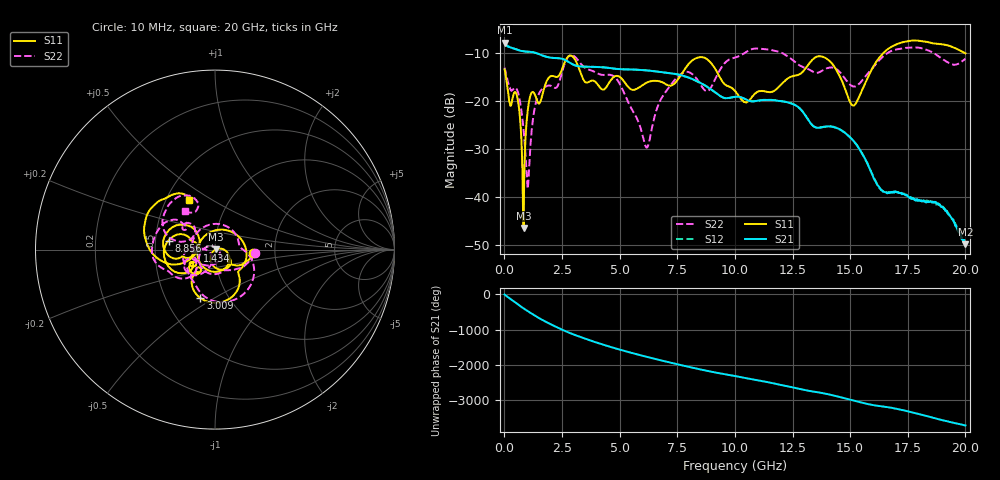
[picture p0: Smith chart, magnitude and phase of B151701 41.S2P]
!  2-Port S-parameters saved by WinCal
! VAR MeasName=S-Parameters (CALIBRATED_DATA) read from VNA (N5244A)
! VAR MeasDate=2015-12-24 19:14:13
! VAR NAME=B151701 41
! VAR FILENAME=B151701 41.S2P
! VAR DATE=2015-12-24 19:14:13
! VAR PHYS_PORTS=1,3
# Hz S DB R 50
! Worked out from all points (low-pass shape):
!   801 points, 10 MHz to 20 GHz, reference 50 ohm
!   highest |S21| = -7.85 dB at 10 MHz (marker M1); lowest = -49.8 dB at 20 GHz (marker M2)
!   |S21| within 3 dB of the highest: start of sweep to 1.852 GHz
!   lowest |S11| = -46.4 dB at 834.6 MHz (marker M3), VSWR 1.01, Z = 50.5 + j0.0707 ohm
!   |S11| at or under -10 dB: start of sweep to 16.45 GHz; 19.97049 GHz to end of sweep
!   |S22| runs from -38.2 to -8.9 dB; largest |S21 - S12| = 0.0028
!   S11 on the Smith chart (normalised r, x): 10 MHz: 1.54, -0.06; 1.434 GHz: 0.82, -0.01; 3.009 GHz: 0.74, -0.43; 8.856 GHz: 0.59, +0.06; 20 GHz: 0.65, +0.40
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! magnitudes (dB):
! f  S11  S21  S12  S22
! 10 MHz  -13.4  -7.8  -7.8  -13.1
! 234.9 MHz  -20.4  -8.8  -8.8  -17.2
! 559.7 MHz  -19.2  -9.4  -9.3  -17.8
! 834.6 MHz  -46.4  -9.7  -9.7  -26.1
! 1.034 GHz  -21.1  -9.8  -9.7  -37.2
! 1.434 GHz  -20.1  -10.1  -10.1  -19.2
! 3.009 GHz  -11.0  -12.5  -12.5  -10.6
! 3.358 GHz  -14.8  -12.8  -12.8  -12.5
! 4.283 GHz  -17.6  -13.0  -13.0  -14.6
! 4.883 GHz  -14.8  -13.3  -13.3  -15.5
! 6.157 GHz  -16.2  -13.6  -13.6  -29.7
! 6.682 GHz  -15.9  -13.9  -13.9  -20.7
! 7.806 GHz  -13.5  -14.8  -14.8  -14.0
! 8.856 GHz  -11.6  -17.2  -17.2  -17.8
! 10.01 GHz  -17.9  -19.1  -19.1  -11.0
! 11.65 GHz  -18.0  -19.8  -19.8  -9.5
! 13.35 GHz  -11.5  -25.0  -25.0  -13.8
! 14.15 GHz  -11.9  -25.3  -25.2  -13.0
! 15.15 GHz  -21.0  -28.4  -28.4  -17.0
! 16.68 GHz  -9.1  -39.0  -38.9  -9.9
! 18.95 GHz  -8.2  -42.0  -41.7  -11.1
! 20 GHz  -10.1  -49.8  -50.1  -11.2
